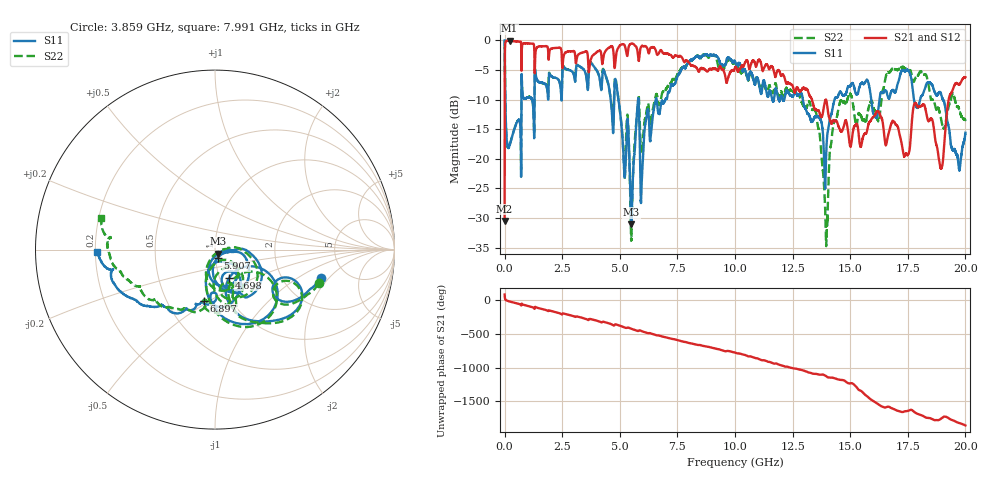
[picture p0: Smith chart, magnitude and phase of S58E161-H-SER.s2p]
!{S58E161}
!Johanson Technology Inc.
!www.johansontechnology.com
!Test Board Conditions:
!Substrate Type  RO4350B
!Substrate Thickness  60 mil
!Substrate Dk  3.66
!TL Type: GCPW
!TL Trace Width  115 mil
!TL Gap  52 mil
!Electrode orientation  Horizontal
!DUT TOPOLOGY	SERIES
!Mounting Pad LxW  55x428 mil
! Created Wed Apr 14 11:23:23 2021
# mhz S ma R 50
! 2 Port Network Data from SP1.SP block
! freq  magS11  angS11  magS21  angS21  magS12  angS12  magS22  angS22
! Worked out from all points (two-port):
!   20001 points, 300 kHz to 20 GHz, reference 50 ohm
!   highest |S21| = -0.08 dB at 213.3 MHz (marker M1); lowest = -30.5 dB at 300 kHz (marker M2)
!   |S21| within 3 dB of the highest: 4.819 GHz to 5.804 GHz (984.4 MHz wide, 18.5 % of centre); 5.841 GHz to 7.722 GHz (1.881 GHz wide, 27.7 % of centre)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
!   lowest |S11| = -31.1 dB at 5.501 GHz (marker M3), VSWR 1.06, Z = 51.6 - j2.36 ohm
!   |S11| at or under -10 dB: 4.938 GHz to 5.793 GHz (855.2 MHz wide, 15.9 % of centre); 12.95 GHz to 14.32 GHz (1.377 GHz wide, 10.1 % of centre); 19.03 GHz to end of sweep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
!   |S22| runs from -34.8 to 0.0 dB; largest |S21 - S12| = 0.0095
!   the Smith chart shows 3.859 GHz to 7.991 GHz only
!   S11 on the Smith chart (normalised r, x): 3.859 GHz: 3.22, -1.63; 4.698 GHz: 1.12, -0.36; 5.907 GHz: 1.02, -0.09; 6.897 GHz: 0.75, -0.47; 7.991 GHz: 0.21, -0.01
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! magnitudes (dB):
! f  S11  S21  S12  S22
! 300 kHz  0.0  -30.5  -30.5  0.0
! 102.3 MHz  -17.3  -0.1  -0.1  -17.3
! 213.3 MHz  -17.7  -0.1  -0.1  -17.7
! 3.334 GHz  -4.6  -2.1  -2.1  -4.6
! 3.859 GHz  -4.3  -2.4  -2.5  -4.3
! 4.698 GHz  -15.1  -1.3  -1.3  -14.2
! 5.342 GHz  -13.4  -2.3  -2.3  -12.9
! 5.501 GHz  -31.1  -0.6  -0.5  -33.7
! 5.758 GHz  -11.6  -1.6  -1.6  -11.7
! 5.907 GHz  -26.3  -1.2  -1.2  -17.8
! 6.667 GHz  -12.2  -2.3  -2.4  -10.5
! 6.897 GHz  -10.6  -2.2  -2.2  -8.7
! 7.991 GHz  -3.7  -3.7  -3.7  -3.6
! 10 GHz  -3.6  -4.6  -4.6  -3.8
! 13.33 GHz  -13.8  -10.0  -10.1  -11.7
! 13.96 GHz  -19.0  -10.1  -10.2  -34.6
! 14.56 GHz  -8.7  -15.1  -15.0  -10.5
! 16.21 GHz  -12.0  -12.0  -12.1  -13.6
! 16.67 GHz  -9.8  -15.7  -15.8  -5.4
! 18.16 GHz  -9.0  -10.8  -10.8  -5.7
! 18.95 GHz  -9.1  -21.6  -21.6  -13.5
! 20 GHz  -15.6  -6.2  -6.3  -13.5
